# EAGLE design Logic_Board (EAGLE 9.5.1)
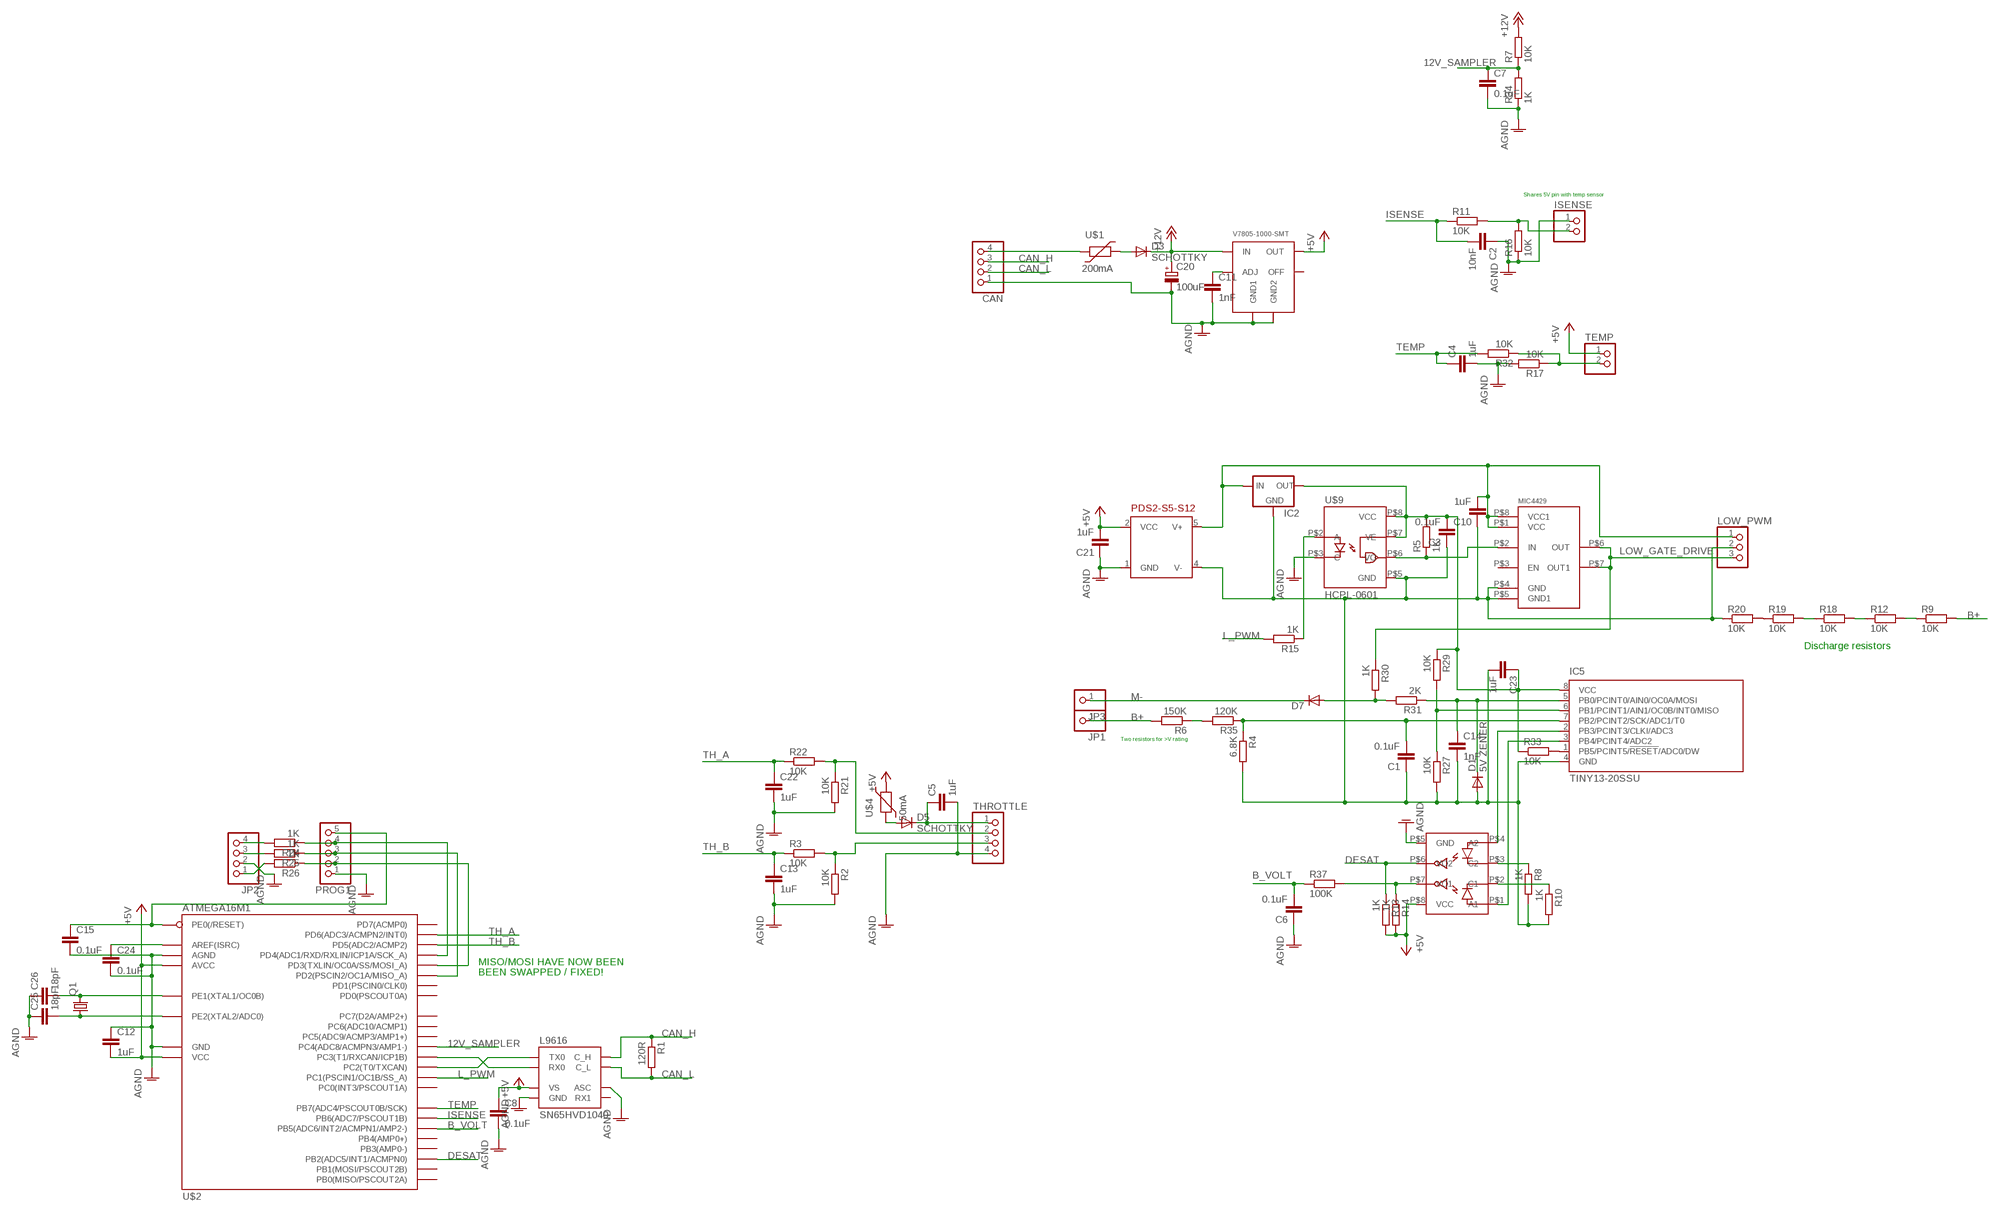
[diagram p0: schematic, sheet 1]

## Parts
C1  0.1uF  C-EUC1206  [C1206]
C2  10nF  C-EUC1206  [C1206]
C3  0.1uF  C-EUC1206  [C1206]
C4  1uF  C-EUC1206  [C1206]
C5  1uF  C-EUC1206  [C1206]
C6  0.1uF  C-EUC1206  [C1206]
C7  0.1uF  C-EUC1206  [C1206]
C8  0.1uF  C-EUC1206  [C1206]
C10  1uF  C-EUC1206  [C1206]
C11  1nF  C-EUC1206  [C1206]
C12  1uF  C-EUC1206  [C1206]
C13  1uF  C-EUC1206  [C1206]
C14  1nF  C-EUC1206  [C1206]
C15  0.1uF  C-EUC1206  [C1206]
C20  100uF  CPOL-EUD  [PANASONIC_D]
C21  1uF  C-EUC1206  [C1206]
C22  1uF  C-EUC1206  [C1206]
C23  1uF  C-EUC1206  [C1206]
C24  0.1uF  C-EUC1206  [C1206]
C25  18pF  C-EUC1206  [C1206]
C26  18pF  C-EUC1206  [C1206]
CAN  PINHD-1X4  [1X04]
D1  5V ZENER  DIODE-SOD123  [SOD123]
D3  SCHOTTKY  DIODE-SOD123  [SOD123]
D5  SCHOTTKY  DIODE-SOD123  [SOD123]
D7  DIODE-SOD123  [SOD123]
IC2  78LXXSOT89  [SOT89R]
IC5  TINY13-20SSU  [8S1]
ISENSE  PINHD-1X2  [1X02]
JP1  PINHD-1X1  [1X01]
JP2  PINHD-1X4  [1X04]
JP3  PINHD-1X1  [1X01]
LOW_PWM  PINHD-1X3  [1X03]
MIC4429  IXDD414CI  [SOIC8]
PDS2-S5-S12  PDS2  [PDS2]
PROG1  PINHD-1X5  [1X05]
Q1  CRYSTALHC49UP  [HC49UP]
R1  120R  R-EU_R1206  [R1206]
R2  10K  R-EU_R1206  [R1206]
R3  10K  R-EU_R1206  [R1206]
R4  6.8K  R-EU_R1206  [R1206]
R5  1K  R-EU_R1206  [R1206]
R6  150K  R-EU_R1206  [R1206]
R7  10K  R-EU_R1206  [R1206]
R8  1K  R-EU_R1206  [R1206]
R9  10K  R-EU_R1206  [R1206]
R10  1K  R-EU_R1206  [R1206]
R11  10K  R-EU_R1206  [R1206]
R12  10K  R-EU_R1206  [R1206]
R13  1K  R-EU_R1206  [R1206]
R14  1K  R-EU_R1206  [R1206]
R15  1K  R-EU_R1206  [R1206]
R16  10K  R-EU_R1206  [R1206]
R17  10K  R-EU_R1206  [R1206]
R18  10K  R-EU_R1206  [R1206]
R19  10K  R-EU_R1206  [R1206]
R20  10K  R-EU_R1206  [R1206]
R21  10K  R-EU_R1206  [R1206]
R22  10K  R-EU_R1206  [R1206]
R24  1K  R-EU_R1206  [R1206]
R25  1K  R-EU_R1206  [R1206]
R26  1K  R-EU_R1206  [R1206]
R27  10K  R-EU_R1206  [R1206]
R29  10K  R-EU_R1206  [R1206]
R30  1K  R-EU_R1206  [R1206]
R31  2K  R-EU_R1206  [R1206]
R32  10K  R-EU_R1206  [R1206]
R33  10K  R-EU_R1206  [R1206]
R34  1K  R-EU_R1206  [R1206]
R35  120K  R-EU_R1206  [R1206]
R37  100K  R-EU_R1206  [R1206]
SN65HVD1040  L9616  [SOIC8]
TEMP  PINHD-1X2  [1X02]
THROTTLE  PINHD-1X4  [1X04]
U$1  200mA  1206_POLYSWITCH  [1206]
U$2  ATMEGA16M1  [TQFP32]
U$4  50mA  1206_POLYSWITCH  [1206]
U$7  HCPL-2631SOIC8  [SOIC8]
U$9  HCPL-0601  [SOIC8@1]
V7805-1000-SMT  V78-1000-SMT  [V78-1000-SMT]

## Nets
12V_SAMPLER: C7.1 R7.1 R34.2 U$2.17(PC4(ADC8/ACMPN3/AMP1-))
+5V: C8.1 C12.2 C21.2 PDS2-S5-S12.2(VCC) R13.2 R14.2 SN65HVD1040.P$3(VS) TEMP.1 U$2.4(VCC) U$2.19(AVCC) U$4.P$2 U$7.P$8(VCC) V7805-1000-SMT.5(OUT)
+12V: C20.+ D3.C R7.2 V7805-1000-SMT.1(IN)
AGND: C2.1 C4.2 C5.2 C6.1 C7.2 C8.2 C11.2 C12.1 C13.2 C15.2 C20.- C21.1 C22.2 C24.2 C25.1 C26.1 CAN.1 ISENSE.1 JP2.2 PDS2-S5-S12.1(GND) PROG1.1 R2.2 R16.1 R17.2 R21.2 R34.1 SN65HVD1040.P$2(GND) SN65HVD1040.P$8(ASC) THROTTLE.4 U$2.5(GND) U$2.20(AGND) U$7.P$5(GND) U$9.P$3(C) V7805-1000-SMT.7(GND1) V7805-1000-SMT.9(GND2)
ASDF: C1.1 C3.1 C10.1 C14.2 C23.2 D1.A IC2.4(GND) IC5.4(GND) LOW_PWM.2 MIC4429.P$4(GND) MIC4429.P$5(GND1) PDS2-S5-S12.4(V-) R4.2 R8.2 R10.2 R20.1 R27.2 U$9.P$5(GND)
B+: JP1.1 R6.2 R9.2
B_VOLT: C6.2 R37.1 U$2.26(PB5(ADC6/INT2/ACMPN1/AMP2-))
CAN_H: CAN.3 R1.1 SN65HVD1040.P$7(C_H)
CAN_L: CAN.2 R1.2 SN65HVD1040.P$6(C_L)
DESAT: R13.1 U$2.16(PB2(ADC5/INT1/ACMPN0)) U$7.P$6(VO2)
FDFSD: R17.1 R32.1 TEMP.2
ISENSE: C2.2 R11.1 U$2.27(PB6(ADC7/PSCOUT1B))
L_PWM: R15.2 U$2.3(PC1(PSCIN1/OC1B/SS_A))
LOW_GATE_DRIVE: LOW_PWM.3 MIC4429.P$6(OUT) MIC4429.P$7(OUT1) R30.1
M-: D7.C JP3.1
N$2: C10.2 IC2.1(IN) LOW_PWM.1 MIC4429.P$1(VCC) MIC4429.P$8(VCC1) PDS2-S5-S12.5(V+)
N$3: SN65HVD1040.P$1(TX0) U$2.6(PC2(T0/TXCAN))
N$4: SN65HVD1040.P$4(RX0) U$2.7(PC3(T1/RXCAN/ICP1B))
N$5: PROG1.2 R26.1 U$2.2(PD3(TXLIN/OC0A/SS/MOSI_A))
N$6: R9.1 R12.2
N$7: JP2.1 R26.2
N$8: C1.2 IC5.7(PB2/PCINT2/SCK/ADC1/T0) R4.1 R35.1
N$9: R18.1 R19.2
N$10: R12.1 R18.2
N$11: C5.1 D5.C THROTTLE.1
N$12: R2.1 R3.2 THROTTLE.3
N$13: R19.1 R20.2
N$14: C26.2 Q1.2 U$2.10(PE1(XTAL1/OC0B))
N$15: ISENSE.2 R11.2 R16.2
N$16: C25.2 Q1.1 U$2.11(PE2(XTAL2/ADC0))
N$17: D5.A U$4.P$1
N$18: R8.1 U$7.P$3(C2)
N$21: CAN.4 U$1.P$1
N$22: C24.1 U$2.21(AREF(ISRC))
N$23: R15.1 U$9.P$2(A)
N$25: JP2.4 R24.2
N$26: R6.1 R35.2
N$27: JP2.3 R25.2
N$30: R21.1 R22.2 THROTTLE.2
N$32: MIC4429.P$2(IN) R5.1 U$9.P$6(VO)
N$33: C15.1 PROG1.5 U$2.31(PE0(/RESET))
N$34: PROG1.3 R25.1 U$2.1(PD2(PSCIN2/OC1A/MISO_A))
N$35: C3.2 C23.1 IC2.2(OUT) IC5.8(VCC) R5.2 R29.1 R33.1 U$9.P$7(VE) U$9.P$8(VCC)
N$36: C11.1 V7805-1000-SMT.6(ADJ)
N$37: PROG1.4 R24.1 U$2.12(PD4(ADC1/RXD/RXLIN/ICP1A/SCK_A))
N$38: C14.1 D1.C IC5.5(PB0/PCINT0/AIN0/OC0A/MOSI) R31.1
N$39: D3.A U$1.P$2
N$41: D7.A R30.2 R31.2
N$42: IC5.6(PB1/PCINT1/AIN1/OC0B/INT0/MISO) R27.1 R29.2
N$44: R10.1 U$7.P$2(C1)
N$45: IC5.1(PB5/PCINT5/!RESET!/ADC0/DW) R33.2
N$46: IC5.2(PB3/PCINT3/CLKI/ADC3) U$7.P$4(A2)
N$47: IC5.3(PB4/PCINT4/ADC2) U$7.P$1(A1)
PWM: R14.1 R37.2 U$7.P$7(VO1)
TEMP: C4.1 R32.2 U$2.28(PB7(ADC4/PSCOUT0B/SCK))
TH_A: C22.1 R22.1 U$2.14(PD6(ADC3/ACMPN2/INT0))
TH_B: C13.1 R3.1 U$2.13(PD5(ADC2/ACMP2))
Unconnected: MIC4429.P$3(EN) SN65HVD1040.P$5(RX1) U$2.8(PB0(MISO/PSCOUT2A)) U$2.9(PB1(MOSI/PSCOUT2B)) U$2.15(PD7(ACMP0)) U$2.18(PC5(ADC9/ACMP3/AMP1+)) U$2.22(PC6(ADC10/ACMP1)) U$2.23(PB3(AMP0-)) U$2.24(PB4(AMP0+)) U$2.25(PC7(D2A/AMP2+)) U$2.29(PD0(PSCOUT0A)) U$2.30(PC0(INT3/PSCOUT1A)) U$2.32(PD1(PSCIN0/CLK0)) V7805-1000-SMT.10(OFF)

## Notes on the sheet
- Shares 5V pin with temp sensor
- Discharge resistors
- Two resistors for >V rating
- MISO/MOSI HAVE NOW BEEN
- BEEN SWAPPED / FIXED!

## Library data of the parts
C1-C8 C10-C15 C21-C26 = resistor:C-EU: CAPACITOR, European symbol
C20 = resistor:CPOL-EU: POLARIZED CAPACITOR, European symbol
CAN JP2 THROTTLE = pinhead:PINHD-1X4: PIN HEADER
D1 D3 D5 D7 = diode:DIODE-: DIODE
IC2 = v-reg:78LXX: VOLTAGE REGULATOR
IC5 = atmel:TINY13: 8-bit AVR Microcontroller with 1K Bytes In-System Programmable Flash Source: http://www.atmel.com/dyn/resources/prod_documents/2535S.pdf
ISENSE TEMP = pinhead:PINHD-1X2: PIN HEADER
JP1 JP3 = pinhead:PINHD-1X1: PIN HEADER
LOW_PWM = pinhead:PINHD-1X3: PIN HEADER
MIC4429 = Ians parts:IXDD414CI: IXYS 14A MOSFET driver
PDS2-S5-S12 = Ians parts:PDS2
PROG1 = pinhead:PINHD-1X5: PIN HEADER
Q1 = crystal:CRYSTAL: CRYSTAL
R1-R22 R24-R27 R29-R35 R37 = resistor:R-EU_: RESISTOR, European symbol
SN65HVD1040 = Ians parts:L9616
U$1 U$4 = Ians parts:1206_POLYSWITCH
U$2 = Ians parts:ATMEGA16M1
U$7 = Ians parts:HCPL-2631
U$9 = Ians parts:HCPL-0601
V7805-1000-SMT = Ians parts:V78-1000-SMT

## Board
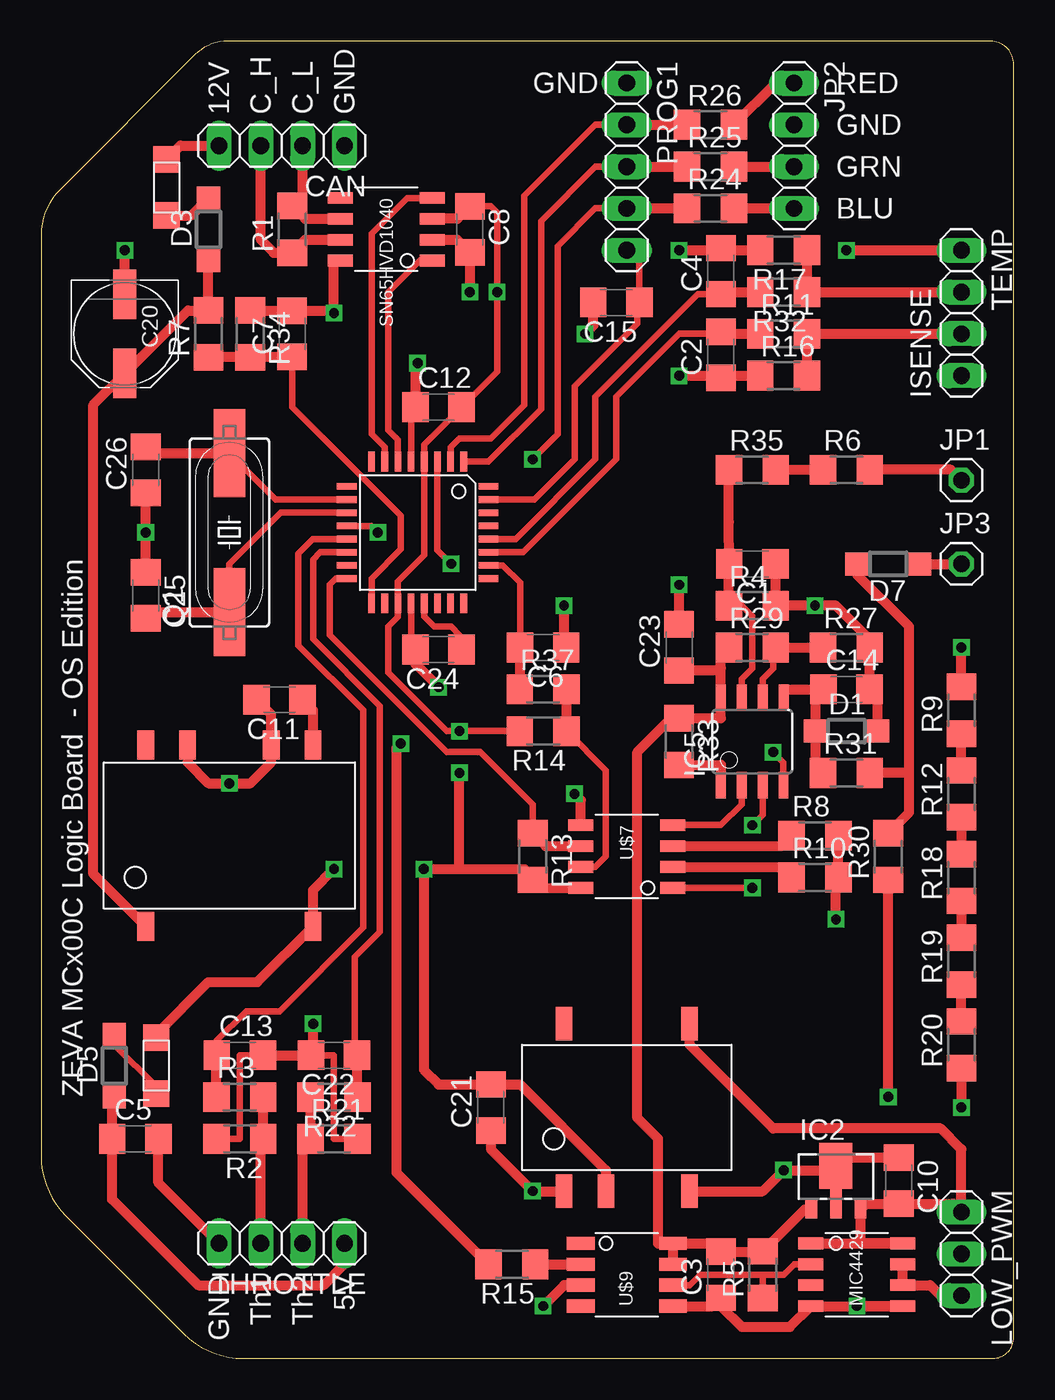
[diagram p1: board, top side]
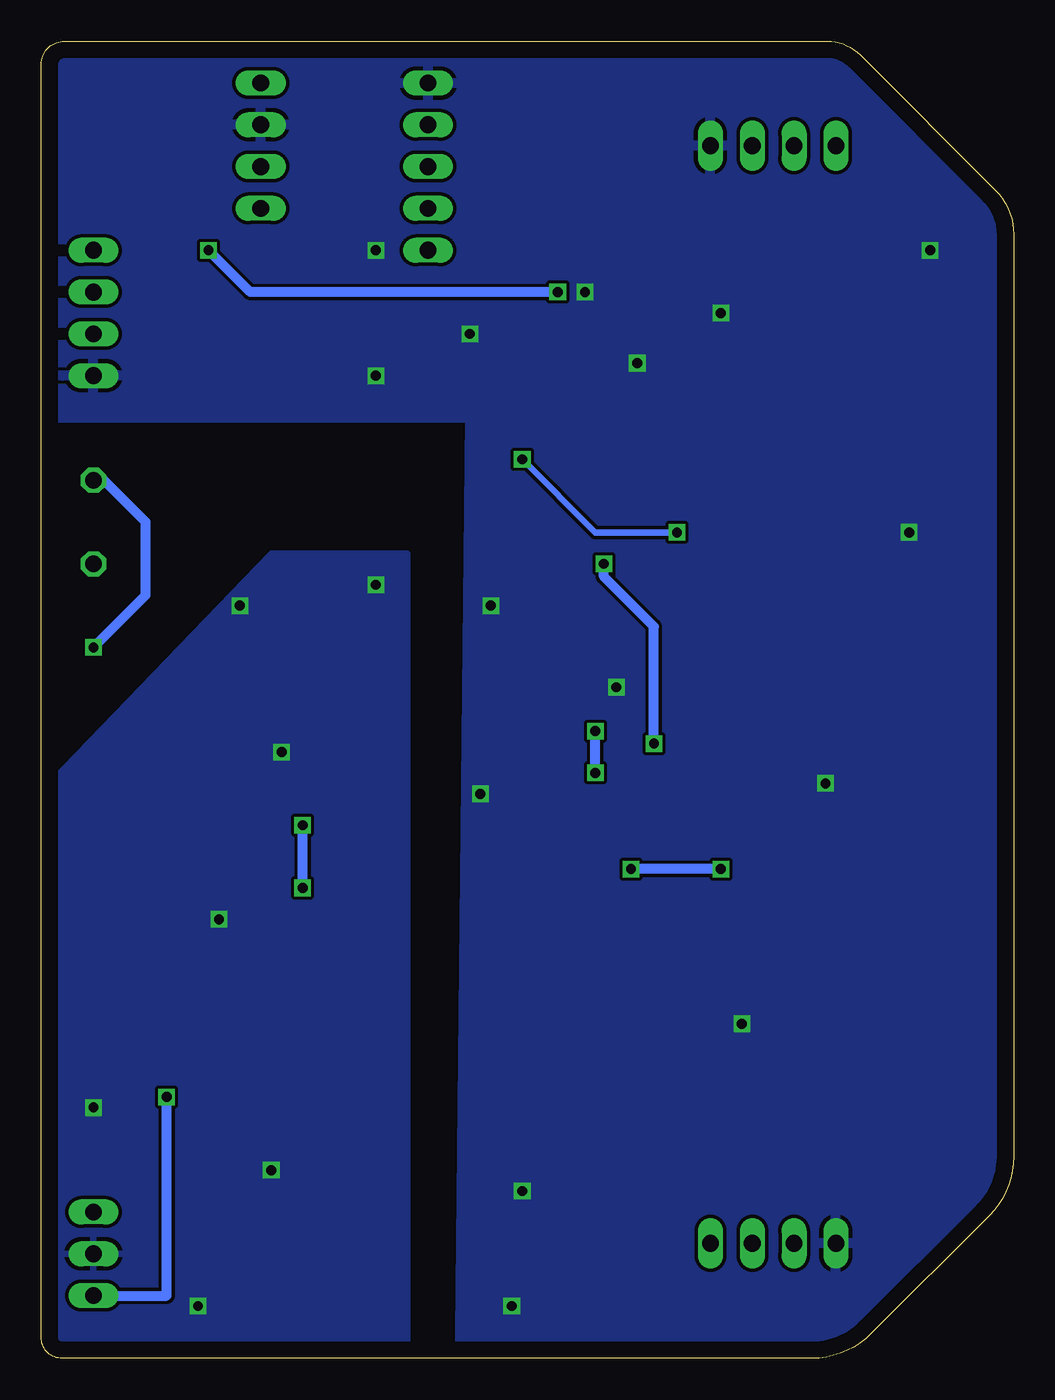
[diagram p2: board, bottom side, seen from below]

Size 59.05 x 80.01 mm. Coordinates in mm from the lower left corner, seen from the top.
Outline: 11.34,80.01 arc45 9.33,79.18 1.12,70.97 arc45 0,68.27 0,12.26 arc45 1.49,8.67 8.67,1.49 arc45 12.26,0 57.78,0 arc90 59.05,1.27 59.05,78.59 arc90 57.63,80.01 11.34,80.01
Copper layers (1*16): Top 0.035mm / dielectric 1.5mm / Bottom 0.035mm
Design rules "default *": minimum track width 10mil, minimum drill 10mil, track to track 8mil, track to pad 8mil, pad to pad 8mil, via to via 8mil, smd to smd 8mil, copper to edge 40mil, drill to drill 8mil, minimum pad ring 10mil, minimum via ring 8mil, stop-mask expansion 4mil, vias tented up to drill 0mil, thermal gap 10mil

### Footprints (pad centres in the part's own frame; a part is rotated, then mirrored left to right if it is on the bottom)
C1206 = smd 1.6 x 1.8: 1 -1.4,0; 2 1.4,0
PANASONIC_D = smd 3 x 1.4: + 2.4,0; - -2.4,0
1X04 = drill 1.016 long: 1 -3.81,0; 2 -1.27,0; 3 1.27,0; 4 3.81,0
SOD123 = smd 1.4 x 1.4: A 1.9,0; C -1.9,0
SOT89R = smd 0.7 x 1.1: 1 1.5,-1.75; 2 -1.5,-1.75 | smd 0.7 x 1.8: 3 0,-1.4 | smd 2 x 2.8: 4 0,0.9
8S1 = smd 0.6 x 1.6: 1 -1.905,-2.654; 2 -0.645,-2.654; 3 0.625,-2.654; 4 1.895,-2.654; 5 1.905,2.654; 6 0.635,2.654; 7 -0.635,2.654; 8 -1.905,2.654
1X02 = drill 1.016 long: 1 -1.27,0; 2 1.27,0
1X01 = drill 1.016 octagon: 1 0,0
1X03 = drill 1.016 long: 1 -2.54,0; 2 0,0; 3 2.54,0
SOIC8 = smd 1.524 x 0.711: P$1 -2.794,1.905; P$2 -2.794,0.635; P$3 -2.794,-0.635; P$4 -2.794,-1.905; P$5 2.794,-1.905; P$6 2.794,-0.635; P$7 2.794,0.635; P$8 2.794,1.905
PDS2 = smd 1.016 x 2.032: 1 -3.81,-5.08; 2 -1.27,-5.08; 4 3.81,-5.08; 5 3.81,5.08; 8 -3.81,5.08
1X05 = drill 1.016 long: 1 -5.08,0; 2 -2.54,0; 3 0,0; 4 2.54,0; 5 5.08,0
HC49UP = smd 5.334 x 1.93: 1 -4.826,0; 2 4.826,0
R1206 = smd 1.6 x 1.803: 1 -1.422,0; 2 1.422,0
1206 = smd 1.6 x 1.6: P$1 -1.7,0; P$2 1.7,0
TQFP32 = smd 1.2 x 0.4: 1 -4.3,2.8; 2 -4.3,2; 3 -4.3,1.2; 4 -4.3,0.4; 5 -4.3,-0.4; 6 -4.3,-1.2; 7 -4.3,-2; 8 -4.3,-2.8; 17 4.3,-2.8; 18 4.3,-2; 19 4.3,-1.2; 20 4.3,-0.4; 21 4.3,0.4; 22 4.3,1.2; 23 4.3,2; 24 4.3,2.8 | smd 0.4 x 1.2: 9 -2.8,-4.3; 10 -2,-4.3; 11 -1.2,-4.3; 12 -0.4,-4.3; 13 0.4,-4.3; 14 1.2,-4.3; 15 2,-4.3; 16 2.8,-4.3; 25 2.8,4.3; 26 2,4.3; 27 1.2,4.3; 28 0.4,4.3; 29 -0.4,4.3; 30 -1.2,4.3; 31 -2,4.3; 32 -2.8,4.3
SOIC8@1 = smd 1.676 x 0.813: P$1 -2.794,1.905; P$2 -2.794,0.635; P$3 -2.794,-0.635; P$4 -2.794,-1.905; P$5 2.794,-1.905; P$6 2.794,-0.635; P$7 2.794,0.635; P$8 2.794,1.905
V78-1000-SMT = smd 1.778 x 1.016: 1 -5.512,5.08; 5 -5.512,-5.08; 6 5.512,-5.08; 7 5.512,-2.54; 9 5.512,2.54; 10 5.512,5.08

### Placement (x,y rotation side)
C1  43.18,48.26 180 top
C2  41.27,60.96 90 top
C3  41.27,5.08 90 top
C4  41.27,66.04 90 top
C5  5.71,13.34 0 top
C6  30.48,43.18 180 top
C7  15.24,62.23 90 top
C8  26.04,68.58 270 top
C10  52.07,10.79 270 top
C11  14.48,40.01 180 top
C12  24.13,57.78 0 top
C13  12.06,18.41 0 top
C14  48.9,40.64 0 top
C15  34.92,64.14 180 top
C20  5.08,62.23 270 top
C21  27.3,15.24 90 top
C22  17.78,18.41 180 top
C23  38.73,43.18 90 top
C24  24.13,43.05 180 top
C25  6.35,46.35 270 top
C26  6.35,53.98 90 top
CAN  14.61,73.66 180 top
D1  48.9,38.1 0 top
D3  10.16,68.58 90 top
D5  4.45,17.78 90 top
D7  51.44,48.26 180 top
IC2  48.26,10.79 0 top
IC5  43.18,37.47 0 top
ISENSE  55.88,60.96 90 top
JP1  55.88,53.34 0 top
JP2  45.72,73.66 270 top
JP3  55.88,48.26 0 top
LOW_PWM  55.88,6.35 270 top
MIC4429  49.53,5.08 0 top
PDS2-S5-S12  35.56,15.24 0 top
PROG1  35.56,72.39 270 top
Q1  11.43,50.16 90 top
R1  15.24,68.58 90 top
R2  12.06,13.34 180 top
R3  12.06,15.88 0 top
R4  43.18,45.72 0 top
R5  43.81,5.08 90 top
R6  48.9,53.98 0 top
R7  10.16,62.23 90 top
R8  46.99,31.75 0 top
R9  55.88,39.37 90 top
R10  46.99,29.21 0 top
R11  45.09,62.23 0 top
R12  55.88,34.29 90 top
R13  29.84,30.48 270 top
R14  30.48,38.1 180 top
R15  28.57,5.71 180 top
R16  45.09,59.69 0 top
R17  45.09,67.31 180 top
R18  55.88,29.21 90 top
R19  55.88,24.13 90 top
R20  55.88,19.05 90 top
R21  17.78,13.34 0 top
R22  17.78,15.88 180 top
R24  40.64,69.85 0 top
R25  40.64,72.39 0 top
R26  40.64,74.93 0 top
R27  48.9,43.18 0 top
R29  43.18,43.18 0 top
R30  51.44,30.48 90 top
R31  48.9,35.56 0 top
R32  45.09,64.77 180 top
R33  38.73,37.47 270 top
R34  12.7,62.23 270 top
R35  43.18,53.98 0 top
R37  30.48,40.64 0 top
SN65HVD1040  20.95,68.58 180 top
TEMP  55.88,66.04 270 top
THROTTLE  14.61,6.99 180 top
U$1  7.62,71.12 270 top
U$2  22.86,50.16 270 top
U$4  6.99,17.78 90 top
U$7  35.56,30.48 180 top
U$9  35.56,5.08 0 top
V7805-1000-SMT  11.43,31.75 90 top

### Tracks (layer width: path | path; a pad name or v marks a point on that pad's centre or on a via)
12V_SAMPLER
  Top 0.406: U$2.17 20.06,47.37 21.84,49.15 21.84,51.18 15.24,57.78 C7.1
  Top 0.61: R7.1 R34.2 15.22,60.81 C7.1
+5V  (via drill 0.6)
  Top 0.406: C8.1 27.3,69.98 27.69,69.6 v27.69,64.77 27.69,59.94 C12.2 23.26,55.52 U$2.4 23.26,48.79 21.66,47.19 U$2.19 21.66,45.03 21.08,44.45 21.08,41.66 24.64,38.1 v25.4,38.1 R14.2
  Top 0.61: SN65HVD1040.P$3 25.27,69.22 C8.1 | v17.78,29.72 16.51,28.45 V7805-1000-SMT.5 13.13,22.86 10.16,22.86 6.99,19.68 U$4.P$2 | v48.9,67.31 TEMP.1 | 30.48,28.57 30.33,28.57 R13.2 | 30.48,28.57 U$7.P$8 | 25.4,29.72 v23.24,29.72 23.24,17.53 24.13,16.64 C21.2 29.08,16.64 34.29,11.43 PDS2-S5-S12.2 | 30.48,28.57 29.34,29.72 25.4,29.72 | 25.4,29.72 v25.4,35.56
  Bottom 0.61: v17.78,29.72 v23.24,29.72 | v27.69,64.77 46.35,64.77 v48.9,67.31 | v25.4,35.56 v25.4,38.1
+12V
  Top 0.61: D3.C R7.2 8.9,63.65 C20.+ 3.17,57.92 3.17,29.41 V7805-1000-SMT.1
AGND  (via drill 0.6)
  Top 0.406: R2.2 12.06,13.34 12.06,18.41 C13.2 | R21.2 17.78,13.34 17.78,18.41 C22.2 | U$2.5 22.46,57.52 C12.1 | U$2.20 22.46,43.32 C24.2
  Top 0.61: v16.51,20.32 16.51,18.55 C22.2 C13.2 | U$9.P$3 31.75,4.45 v30.48,3.17 | R16.1 41.41,59.69 C2.1 41.15,59.69 v38.73,59.69 | R17.2 41.41,67.31 C4.2 41.15,67.31 v38.73,67.31 | U$7.P$5 32.77,33.91 v32.38,34.29 | SN65HVD1040.P$2 25.27,67.94 C8.2 v26.04,64.77 | C20.- v5.08,67.31 | R34.1 15.22,63.65 C7.2 17.65,63.63 v17.78,63.5 17.78,66.67 SN65HVD1040.P$8 | C25.1 v6.35,50.16 C26.1 | V7805-1000-SMT.9 8.89,36.2 10.16,34.92 v11.43,34.92 12.7,34.92 13.97,36.2 V7805-1000-SMT.7 13.97,39.11 C11.2 | C15.2 33.52,62.73 v33.02,62.23 | C6.1 31.75,43.31 v31.75,45.72 | C12.1 22.73,60.32 v22.86,60.45 | v24.13,40.77 22.73,42.17 C24.2 | PDS2-S5-S12.1 v29.84,10.16 27.3,12.7 C21.1 | C5.2 7.12,10.66 THROTTLE.4
  pour Bottom: -1.27,81.92 60.33,81.92 60.96,57.15 33.02,57.15 33.66,-1.27 -1.27,-0.64
ASDF  (via drill 0.6)
  Top 0.406: IC5.4 45.08,36.2 v44.45,36.83
  Top 0.61: R8.2 R10.2 48.26,29.21 v48.26,26.67 | U$9.P$5 40.77,3.17 C3.1 41.27,3.17 42.55,1.91 45.47,1.91 MIC4429.P$4 MIC4429.P$5 v49.53,3.17 | C1.1 44.6,48.24 R4.2 v46.99,45.72 48.26,45.72 50.32,43.66 R27.2 50.32,40.66 C14.2 50.8,40.14 D1.A | C23.2 v38.73,46.99 | C10.1 48.76,12.2 IC2.4 47.99,11.43 v45.09,11.43 43.81,10.16 PDS2-S5-S12.4 | R20.1 v55.88,15.24
  pour Bottom: 36.83,-1.27 36.83,48.9 45.09,48.9 61.59,31.75 60.96,-1.27
B+  (via drill 0.6)
  Top 0.61: JP1.1 55.24,53.98 R6.2 | R9.2 v55.88,43.18
  Bottom 0.61: JP1.1 55.24,53.34 52.7,50.8 52.7,46.35 v55.88,43.18
B_VOLT
  Top 0.406: U$2.26 28.04,48.16 29.08,47.12 C6.2
  Top 0.61: R37.1 29.08,40.66 C6.2
CAN_H
  Top 0.61: CAN.3 13.34,67.94 14.12,67.16 R1.1 16.03,67.94 SN65HVD1040.P$7
CAN_L
  Top 0.61: CAN.2 15.88,70.64 R1.2 16.03,69.22 SN65HVD1040.P$6
DESAT
  Top 0.406: 29.57,31.9 R13.1 29.84,33.66 26.67,36.83 24.64,36.83 17.53,43.94 17.53,46.99 17.9,47.37 U$2.16
  Top 0.61: U$7.P$6 30.63,31.11 R13.1
FDFSD
  Top 0.61: R17.1 R32.1 TEMP.2
ISENSE
  Top 0.406: C2.2 41.15,62.23 38.73,62.23 34.92,58.42 34.92,54.61 29.28,48.97 U$2.27
  Top 0.61: R11.1 41.41,62.23 C2.2
L_PWM  (via drill 0.6)
  Top 0.406: U$2.3 24.06,49.09 v24.89,48.26
  Top 0.61: R15.2 21.59,11.28 21.59,37.08 v21.84,37.34
  Bottom 0.61: v21.84,37.34 21.84,44.45 24.89,47.5 v24.89,48.26
LOW_GATE_DRIVE  (via drill 0.6)
  Top 0.61: MIC4429.P$7 MIC4429.P$6 53.98,4.45 54.61,3.81 LOW_PWM.3 | v51.44,15.88 R30.1
  Bottom 0.61: LOW_PWM.3 51.44,3.81 v51.44,15.88
M-
  Top 0.61: D7.C JP3.1
N$2
  Top 0.61: MIC4429.P$1 MIC4429.P$8 49.76,6.99 IC2.1 50.11,9.39 C10.2 55.38,9.39 LOW_PWM.1 55.88,12.7 54.61,13.97 44.45,13.97 39.37,19.05 PDS2-S5-S12.5
N$3
  Top 0.406: U$2.6 21.66,55.81 21.08,56.39 21.08,64.77 22.99,66.67 SN65HVD1040.P$1
N$4
  Top 0.406: SN65HVD1040.P$4 22.23,70.48 20.07,68.33 20.07,56.13 20.86,55.34 U$2.7
N$5
  Top 0.406: PROG1.2 33.66,74.93 29.34,70.61 29.34,57.91 27.3,55.88 25.4,55.88 24.86,55.34 U$2.2
  Top 0.61: PROG1.2 R26.1
N$6
  Top 0.61: R12.2 R9.1
N$7
  Top 0.61: JP2.1 44.6,77.47 R26.2
N$8
  Top 0.406: IC5.7 42.55,41.27 43.18,41.91 43.18,45.09 42.55,45.72 R4.1
  Top 0.61: R4.1 41.76,48.24 C1.2 41.76,50.82 R35.1
N$9
  Top 0.61: R18.1 R19.2
N$10
  Top 0.61: R12.1 R18.2
N$11
  Top 0.61: D5.C 4.32,15.75 C5.1 4.32,9.65 9.53,4.45 17.14,4.45 18.41,5.71 THROTTLE.1
N$12
  Top 0.61: THROTTLE.3 13.34,13.18 R2.1 R3.2
N$13
  Top 0.61: R20.2 R19.1
N$14
  Top 0.406: U$2.10 14.26,52.16 Q1.2
  Top 0.61: Q1.2 6.73,54.99 C26.2
N$15
  Top 0.61: R16.2 R11.2 ISENSE.2
N$16
  Top 0.406: U$2.11 14.54,51.37 11.43,48.26 Q1.1
  Top 0.61: Q1.1 6.73,45.34 C25.2
N$17
  Top 0.406: U$4.P$1 6.99,16.51 4.45,19.05 D5.A
N$18
  Top 0.61: R8.1 44.93,31.11 U$7.P$3
N$21
  Top 0.61: CAN.4 8.46,73.66 U$1.P$1
N$22
  Top 0.406: U$2.21 23.26,45.07 23.88,44.45 24.89,44.45 25.4,43.94 25.4,43.18 C24.1
N$23
  Top 0.61: R15.1 U$9.P$2
N$25
  Top 0.61: R24.2 JP2.4
N$26
  Top 0.61: R35.2 R6.1
N$27
  Top 0.61: R25.2 JP2.3
N$30
  Top 0.61: R22.2 R21.1 15.88,12.85 THROTTLE.2
N$32
  Top 0.406: U$9.P$6 39.37,4.45 40.01,5.08 43.81,5.08 | 43.81,5.08 45.09,5.08 45.72,5.71 MIC4429.P$2 | 43.81,5.08 R5.1
N$33
  Top 0.406: U$2.31 29.94,52.16 32.38,54.61 32.38,59.05 36.2,62.87 36.2,64 C15.1 36.33,66.55 PROG1.5
N$34
  Top 0.406: PROG1.3 33.66,72.39 30.35,69.09 30.35,57.66 27.16,54.47 U$2.1
  Top 0.61: PROG1.3 R25.1
N$35
  Top 0.61: 41.27,41.91 IC5.8 41.27,38.89 R33.1 38.58,38.73 38.1,38.73 36.2,36.83 36.2,14.61 37.47,13.34 37.47,6.99 U$9.P$8 | 41.27,41.91 41.27,42.7 R29.1 | U$9.P$8 U$9.P$7 | U$9.P$8 40.77,6.99 C3.2 43.18,6.48 | 43.18,6.48 43.79,6.48 R5.2 46.36,9.04 IC2.2 | 43.18,6.48 43.59,6.88 | C23.1 41.15,41.78 41.27,41.91
N$36
  Top 0.61: V7805-1000-SMT.6 16.51,39.37 C11.1
N$37  (via drill 0.6)
  Top 0.406: U$2.12 20.05,50.56 v20.45,50.16 | v29.84,54.61 31.37,56.13 31.37,67.56 33.66,69.85 PROG1.4
  Top 0.61: PROG1.4 R24.1
  Bottom 0.406: v20.45,50.16 25.4,50.16 v29.84,54.61
N$38
  Top 0.61: R31.1 46.99,36.04 D1.C 46.99,40.14 C14.1 45.09,40.64 IC5.5
N$39
  Top 0.61: U$1.P$2 9.1,69.42 D3.A
N$41
  Top 0.61: 52.7,35.56 52.7,33.17 R30.2 | 52.7,35.56 R31.2 | 52.7,35.56 52.7,44.45 49.53,47.62 D7.A
N$42
  Top 0.406: IC5.6 43.81,41.27 44.45,41.91 44.45,43.03 R29.2
  Top 0.61: R29.2 R27.1
N$44
  Top 0.61: R10.1 44.93,29.84 U$7.P$2
N$45
  Top 0.61: R33.2 41.27,36.04 IC5.1
N$46
  Top 0.406: IC5.2 42.53,33.65 41.27,32.38 U$7.P$4
N$47  (via drill 0.6)
  Top 0.406: IC5.3 43.8,33.01 v43.18,32.38 | U$7.P$1 v43.18,28.57
  Bottom 0.61: v43.18,28.57 v43.18,32.38
PWM
  Top 0.406: U$7.P$7 33.66,29.84 34.29,30.48 34.29,35.71 R14.1
  Top 0.61: R14.1 R37.2
TEMP
  Top 0.406: 41.15,64.77 C4.1 39.88,64.64 33.66,58.42 33.66,54.61 28.81,49.77 U$2.28
  Top 0.61: R32.2 41.41,64.77 C4.1
TH_A
  Top 0.406: C22.1 19.05,18.55 19.05,24.38 20.57,25.91 20.57,39.62 16.51,43.69 16.51,48.51 16.96,48.97 U$2.14
  Top 0.61: R22.1 19.2,18.39 C22.1
TH_B
  Top 0.406: C13.1 10.67,19.3 12.45,21.08 14.48,21.08 19.56,26.16 19.56,39.37 15.62,43.31 15.62,48.9 16.49,49.77 U$2.13
  Top 0.61: R3.1 10.64,18.39 C13.1

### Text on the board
tPlace: GND | RED | 12V | C_H | C_L | GND | GND | GRN | BLU | ZEVA MCx00C Logic Board - OS Edition | GND | Th1 | Th2 | 5V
